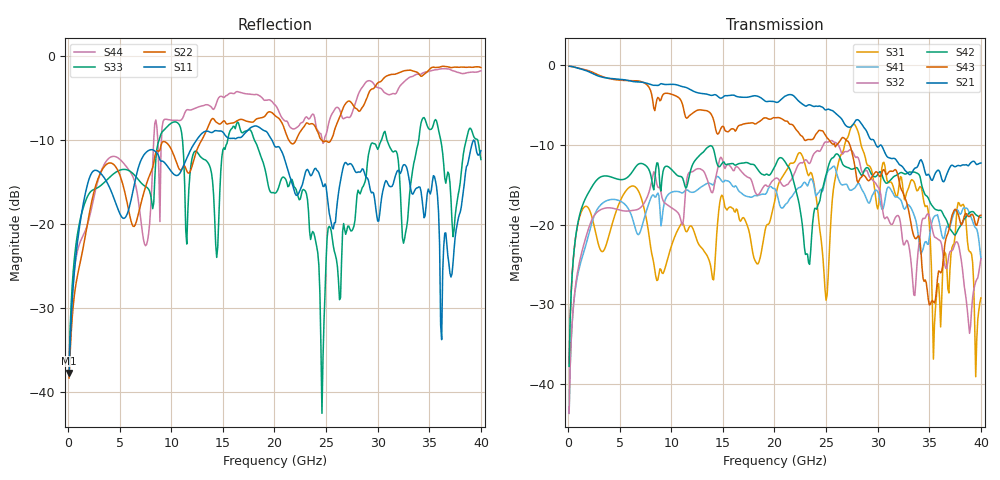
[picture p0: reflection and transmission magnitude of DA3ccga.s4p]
! ADC12DJ3200QML-SP
! 196-pin NWE package
! CCGA Ceramic Package with columns (ceramic column grid array)
! Texas Instruments 4/21/2021
! Single-ended  S-parameters
! PORT#  PORT_NAME  NET_NAME
! PORT1:  DAxN.DIEBUMP DAxN
! PORT2:  DAxN.BGA  DAxN
! PORT3:  DAxP.DIEBUMP DAxP
! PORT4:  DAxP.BGA  DAxP
! Touchstone Ver. 1.0
! Number of ports is 4
# Hz	S	MA	R	50.000000
! SCATTERING PARAMETERS  :
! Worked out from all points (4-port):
!   400 points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, 100 MHz to 40 GHz, reference 50 ohm
!   strongest paths, dB at 100 MHz, 10.1 GHz, 20.1 GHz, 30.1 GHz, 40 GHz:
!     S21: -0.1, -2.4, -4.6, -10.2, -12.2
!     S43: -0.1, -3.6, -6.6, -13.8, -18.8
!     S42: -37.8, -13.2, -12.5, -13.5, -19.1
!     S32: -43.7, -17.9, -14.2, -15.4, -24.3
!     S41: -43.7, -15.9, -15.6, -16.1, -24.2
!     S31: -37.7, -22.3, -16.5, -17.5, -29.2
!   lowest |S11| = -37.8 dB at 100 MHz (marker M1), VSWR 1.03, Z = 51.1 + j0.72 ohm
!   |S11| at or under -10 dB: start of sweep to 12.46 GHz; 19.74 GHz to end of sweep
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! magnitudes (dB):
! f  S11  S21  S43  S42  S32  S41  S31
! 100 MHz  -37.8  -0.1  -0.1  -37.8  -43.7  -43.7  -37.7
! 8.3 GHz  -11.2  -2.5  -5.4  -15.6  -13.3  -16.3  -24.8
! 23 GHz  -13.9  -5.1  -9.4  -23.7  -11.8  -14.7  -12.6
! 24.6 GHz  -15.1  -5.2  -8.2  -15.6  -10.3  -15.9  -22.8
! 29.4 GHz  -16.3  -9.3  -14.1  -13.7  -14.3  -16.6  -13.1
! 36.2 GHz  -33.8  -14.2  -25.9  -18.3  -22.5  -21.2  -29.5
! 40 GHz  -11.3  -12.2  -18.8  -19.1  -24.3  -24.2  -29.2
